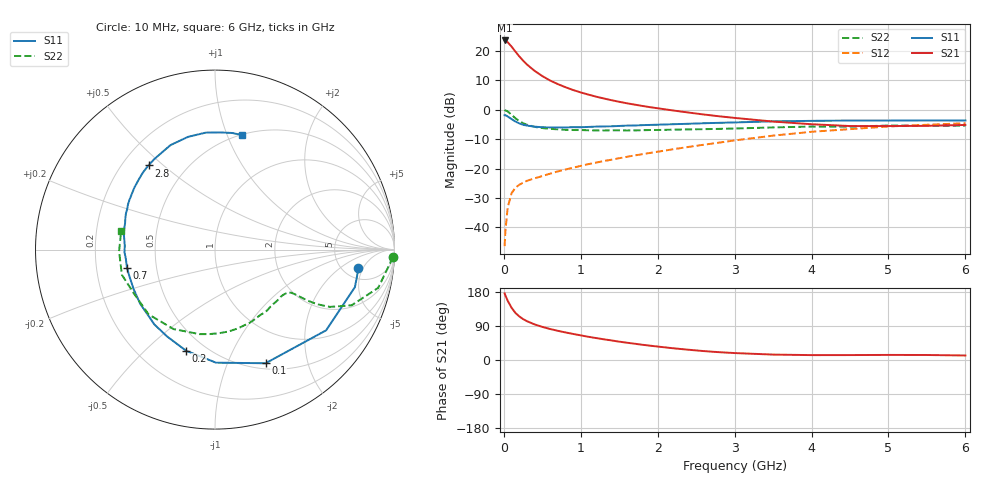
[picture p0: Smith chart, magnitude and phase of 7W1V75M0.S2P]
! Infineon Technologies  Discrete & RF Semiconductors
! BFS17W
! Si NPN RF Bipolar Junction Transistor in SOT323
! VCE = 1.75 V  IC = 5 mA
! Common Emitter S-Parameters:  August  1999
# GHz  S  MA  R  50
!  f  S11  S21  S12  S22
! GHz  MAG  ANG  MAG  ANG  MAG  ANG  MAG  ANG
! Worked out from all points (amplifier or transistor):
!   36 points, 10 MHz to 6 GHz, reference 50 ohm
!   highest |S21| = 23.5 dB at 10 MHz (marker M1)
!   |S21| within 3 dB of that: start of sweep to 127.4 MHz
!   unconditionally stable (mu >= 1): 523.2 MHz to end of sweep
!   at 250 MHz: K = 0.60, MSG = 20.8 dB, |S12| = -24.8 dB
!   at 1.4 GHz: K = 1.29, MAG = 6.9 dB, |S12| = -17.0 dB
!   at 6 GHz: K = 1.10, MAG = -2.2 dB, |S12| = -4.6 dB
!   S11 on the Smith chart (normalised r, x): 10 MHz: 6.87, -4.07; 100 MHz: 0.57, -1.38; 200 MHz: 0.39, -0.68; 700 MHz: 0.34, -0.09; 2.8 GHz: 0.31, +0.45; 6 GHz: 0.51, +1.13
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0.01  0.8062 -7.4  14.99 175.7  0.0048 84.5  0.9916 -2.4
0.02  0.8072 -15.0  14.83 170.3  0.0087 86.2  0.9718 -5.5
0.05  0.7652 -36.0  14.02 156.4  0.0217 72.9  0.9338 -13.2
0.1  0.6931 -66.0  11.81 138.0  0.038 59.6  0.8216 -22.2
0.15  0.63 -89.5  9.724 124.4  0.0472 51.9  0.7156 -26.5
0.2  0.5859 -106.0  8.069 115.1  0.053 48.5  0.6428 -28.2
0.25  0.5527 -118.9  6.811 108.0  0.0573 46.0  0.5899 -28.8
0.3  0.5367 -129.0  5.862 102.5  0.0618 46.1  0.555 -29.0
0.4  0.5145 -144.2  4.567 93.9  0.0683 46.3  0.5102 -29.2
0.5  0.5038 -154.4  3.725 87.4  0.0744 47.9  0.4873 -29.5
0.6  0.4996 -162.3  3.136 81.9  0.0818 49.8  0.473 -30.5
0.7  0.5007 -168.5  2.726 77.1  0.0892 51.8  0.4633 -31.9
0.9  0.5046 -178.4  2.158 68.8  0.1032 54.4  0.4508 -35.8
1.1  0.5091 173.3  1.802 61.2  0.1188 56.4  0.4468 -40.6
1.3  0.5196 166.3  1.549 54.6  0.1342 57.8  0.4431 -46.2
1.6  0.5362 157.6  1.284 45.6  0.158 59.4  0.4433 -54.8
2.2  0.5664 142.6  0.969 31.0  0.2125 60.9  0.4574 -73.9
2.8  0.5977 128.3  0.772 20.6  0.276 59.3  0.472 -94.0
3.5  0.6328 113.1  0.628 14.3  0.3623 54.4  0.4993 -117.5
4.5  0.6537 94.6  0.527 13.0  0.4675 42.6  0.5136 -151.4
5.5  0.6568 81.6  0.532 13.2  0.554 30.8  0.5345 -179.0
6  0.6554 76.5  0.55 11.9  0.5885 25.1  0.5331 168.8
